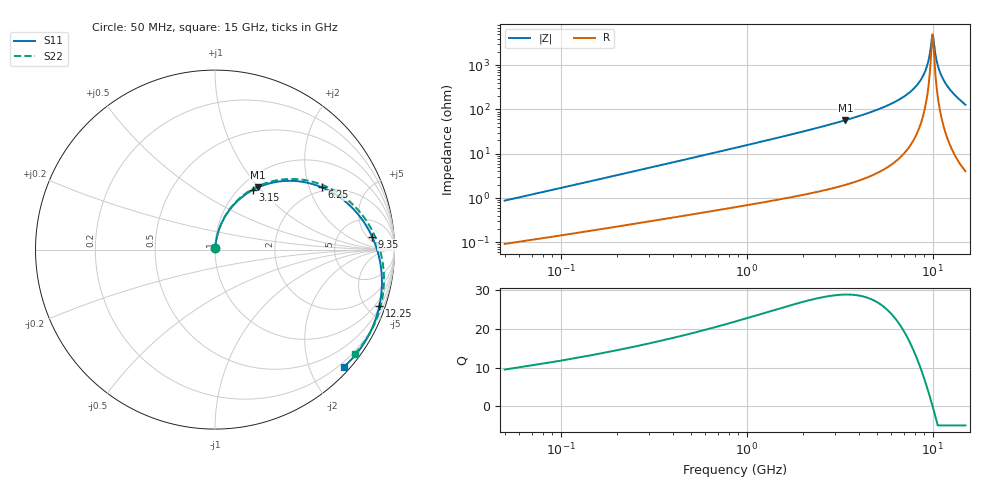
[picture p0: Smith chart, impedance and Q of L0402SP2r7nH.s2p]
!	AVX Thin Film Operation
!	Date:		5 January 2004
!	Description: 	Accu-L®  L0402 Series Thin Film RF Inductors
!	Part Number:	L04022R7AHLTR
!	50 MHz-20GHz Serial Measurements
#	mhz	S	db	R	50
!	S11	S11	S21	S21	S12	S12	S22	S22
!	dB	Phase	dB	Phase	dB	Phase	dB	Phase
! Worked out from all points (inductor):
!   300 points, 50 MHz to 15 GHz, reference 50 ohm
!   read as 1/Y11, port 2 shorted: L = 2.62 nH near 100 MHz
!   highest Q = 28.9 at 3.4 GHz (marker M1), where L = 2.68 nH
!   self-resonance near 9.95 GHz
!   S11 on the Smith chart (normalised r, x): 50 MHz: 1.00, +0.02; 3.15 GHz: 1.15, +0.91; 6.25 GHz: 1.84, +2.43; 9.35 GHz: 11, +7; 12.25 GHz: 0.59, -5.92; 15 GHz: 0.11, -2.58
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50  -42.15 82.7  -0.01 -0.6  -0.01 -0.6  -42.15 82.7
100  -36.50 83.5  -0.01 -1.1  -0.01 -1.1  -36.50 83.5
150  -33.17 83.6  -0.02 -1.6  -0.02 -1.6  -33.17 83.6
250  -28.95 83.2  -0.03 -2.6  -0.03 -2.6  -28.95 83.3
400  -25.04 82.2  -0.04 -4.0  -0.04 -4.0  -25.04 82.3
650  -21.00 80.2  -0.08 -6.5  -0.08 -6.5  -21.00 80.4
1400  -14.62 73.6  -0.23 -13.7  -0.23 -13.7  -14.62 74.0
2550  -9.75 63.0  -0.60 -24.4  -0.60 -24.4  -9.75 63.8
3150  -8.10 57.6  -0.87 -29.8  -0.87 -29.8  -8.10 58.5
3400  -7.51 55.3  -1.00 -32.1  -1.00 -32.1  -7.51 56.3
5050  -4.64 40.7  -2.05 -46.6  -2.05 -46.6  -4.64 42.1
6250  -3.25 30.4  -3.08 -56.7  -3.08 -56.7  -3.25 32.2
7550  -2.16 19.5  -4.49 -67.2  -4.49 -67.2  -2.16 21.7
9350  -1.12 4.7  -7.18 -81.2  -7.18 -81.2  -1.12 7.5
10050  -0.84 -1.0  -8.58 -86.3  -8.58 -86.3  -0.84 2.1
11300  -0.46 -11.2  -11.97 -94.9  -11.97 -94.9  -0.46 -7.6
12250  -0.28 -19.0  -16.06 -100.0  -16.06 -100.0  -0.28 -14.9
12550  -0.24 -21.5  -17.91 -100.7  -17.91 -100.7  -0.24 -17.2
13200  -0.19 -26.9  -24.22 -96.5  -24.22 -96.5  -0.18 -22.3
13750  -0.17 -31.5  -34.34 -31.1  -34.34 -31.1  -0.17 -26.7
14350  -0.19 -36.6  -23.58 39.0  -23.58 39.0  -0.19 -31.4
15000  -0.26 -42.3  -17.39 42.2  -17.39 42.2  -0.25 -36.6
